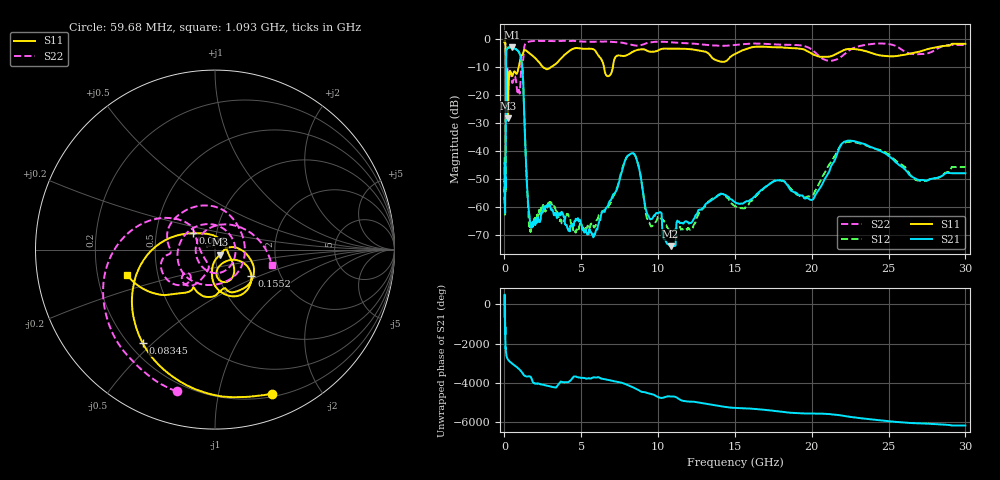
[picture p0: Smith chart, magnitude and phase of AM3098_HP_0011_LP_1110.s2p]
! Date/Time: Thu, Feb 28, 2019 8:34 AM
! Network Analyzer: Agilent Technologies E8364B Rev: A.07.50.67
! Sweep from 0.010 to 30.000 GHz, 1601 Points, Sweep Type: LOG
! Power Supply: 5.022 V, 0.002 A
# Hz S DB R 50
!freq MagS11 AngS11 MagS21 AngS21 MagS12 AngS12 MagS22 AngS22
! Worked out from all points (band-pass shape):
!   1601 points, 10 MHz to 30 GHz, reference 50 ohm
!   highest |S21| = -2.79 dB at 498 MHz (marker M1); lowest = -74.0 dB at 10.81 GHz (marker M2)
!   |S21| within 3 dB of the highest: 108.9 MHz to 1.028 GHz (919.1 MHz wide, 162 % of centre)
!   lowest |S11| = -28.2 dB at 232.8 MHz (marker M3), VSWR 1.08, Z = 52.8 - j2.9 ohm
!   |S11| at or under -10 dB: 93.01 MHz to 922.2 MHz (829.2 MHz wide, 163 % of centre); 2.532 GHz to 2.997 GHz (464.4 MHz wide, 16.8 % of centre); 6.487 GHz to 7.053 GHz (566.5 MHz wide, 8.37 % of centre)
!   |S22| runs from -22.5 to -0.5 dB; largest |S21 - S12| = 0.011
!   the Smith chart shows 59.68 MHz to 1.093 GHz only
!   S11 on the Smith chart (normalised r, x): 59.68 MHz: 0.23, -1.45; 83.45 MHz: 0.25, -0.47; 96 MHz: 0.77, +0.14; 155.2 MHz: 1.42, -0.45; 1.093 GHz: 0.33, -0.13
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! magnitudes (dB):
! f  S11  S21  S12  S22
! 10 MHz  -0.4  -44.1  -42.1  -0.6
! 38.04 MHz  -0.5  -60.6  -60.7  -1.0
! 59.68 MHz  -1.3  -49.8  -53.6  -1.7
! 73.27 MHz  -2.0  -53.0  -51.3  -2.5
! 83.45 MHz  -3.6  -36.5  -36.2  -4.0
! 96 MHz  -16.2  -12.4  -12.4  -20.3
! 144.7 MHz  -15.3  -3.6  -3.5  -13.1
! 155.2 MHz  -12.0  -3.5  -3.5  -11.3
! 232.8 MHz  -28.2  -2.9  -2.9  -12.0
! 309.6 MHz  -12.5  -2.9  -2.8  -11.2
! 498 MHz  -13.1  -2.8  -2.8  -15.4
! 550.5 MHz  -12.5  -3.0  -2.9  -15.1
! 1.093 GHz  -5.9  -7.4  -7.4  -9.7
! 1.606 GHz  -4.8  -62.4  -66.0  -0.8
! 2.084 GHz  -7.1  -65.8  -64.5  -0.5
! 5.812 GHz  -3.6  -70.6  -67.0  -0.8
! 7.926 GHz  -5.7  -42.3  -42.4  -1.5
! 10.81 GHz  -3.3  -74.0  -68.8  -1.0
! 13.88 GHz  -7.6  -56.0  -55.9  -2.2
! 19.9 GHz  -4.8  -57.4  -56.3  -3.3
! 22.67 GHz  -3.4  -36.3  -36.7  -3.2
! 30 GHz  -1.6  -47.9  -45.7  -2.0
